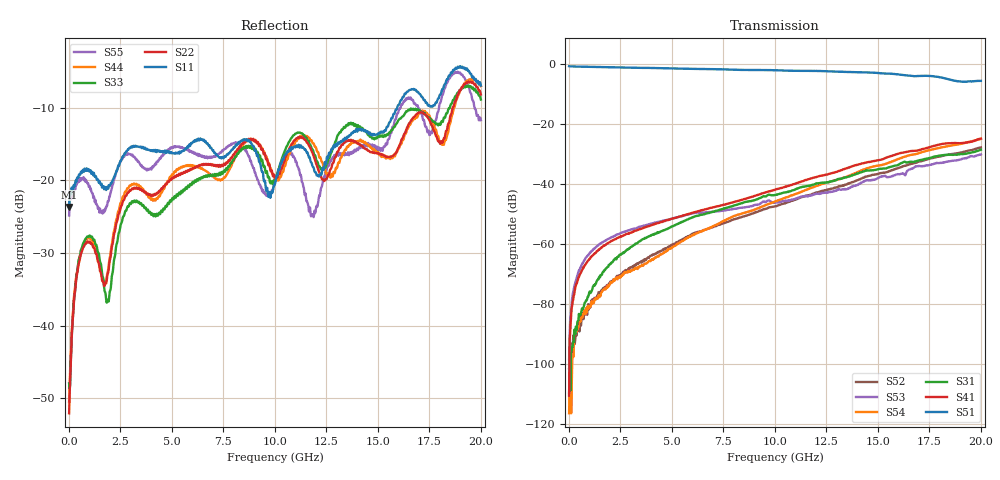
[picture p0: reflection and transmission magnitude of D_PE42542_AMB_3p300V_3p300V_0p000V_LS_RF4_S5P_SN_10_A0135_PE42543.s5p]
! Device ID: PE42542
! Device ID: PE42542
! File Path: z:\PE42542\PE42543_20140723_inv\AMB\3p300\LS_RF4\PE42542_AMB_3p300V_3p300V_0p000V_LS_RF4_S5P_SN_10_A0135_PE42543.s5p
! Serial: 10
! Lot: A0135_PE42543
! Temp: AMB
! VDD: 3.300
! VSS: 0.000
! Control_Hi: 3.300
! Control_Lo: 0.000
! Logic State: LS_RF4
! Port 1: RFC
! Port 2: RF1
! Port 3: RF2
! Port 5: RF3
! Port 6: RF4
! ThroughPath:1-6
! IDD: -0.000135342697
! ISS: 1.01285291e-009
#  Hz  S  RI  R  50
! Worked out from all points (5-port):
!   801 points, 10 MHz to 20 GHz, reference 50 ohm
!   strongest paths, dB at 10 MHz, 5.008 GHz, 10.01 GHz, 15 GHz, 20 GHz:
!     S51: -0.7, -1.5, -2.1, -3.0, -5.6
!     S41: -110.6, -51.6, -41.9, -32.1, -24.9
!     S31: -109.7, -54.1, -43.7, -35.1, -28.6
!     S54: -116.4, -61.3, -45.8, -33.9, -25.0
!     S53: -98.5, -51.6, -46.2, -38.0, -30.2
!     S52: -101.5, -60.3, -47.4, -36.6, -27.8
!   lowest |S11| = -23.7 dB at 10 MHz (marker M1), VSWR 1.14, Z = 56.8 - j1.79 ohm
!   |S11| at or under -10 dB: start of sweep to 15.94 GHz
